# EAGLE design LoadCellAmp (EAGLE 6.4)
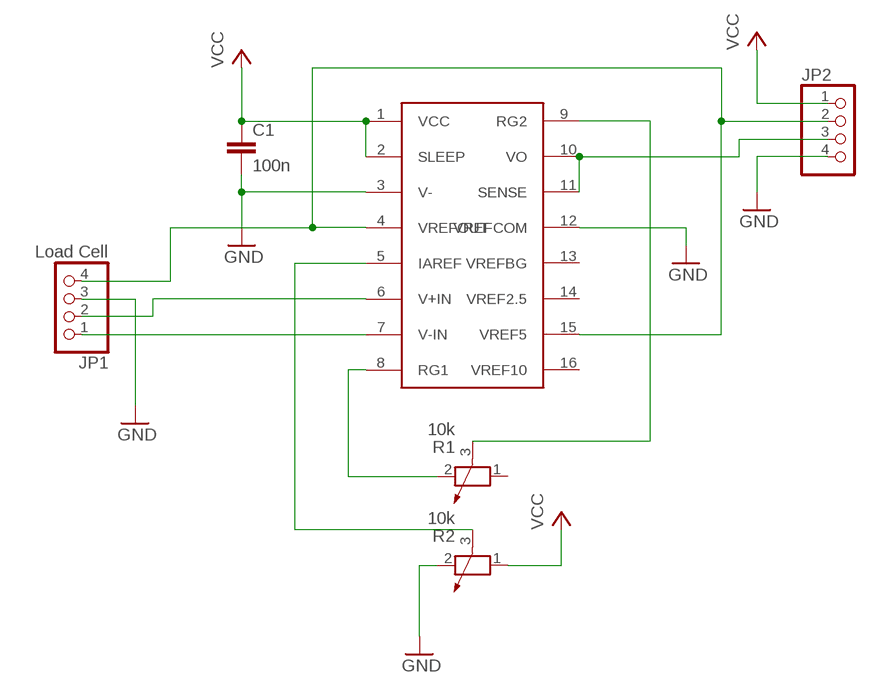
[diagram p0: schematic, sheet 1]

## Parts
C1  100n  C-EUC0603  [C0603]
JP1  Load Cell  PINHD-1X4  [1X04]
JP2  PINHD-1X4  [1X04]
R1  10k  POTENTIOMETER_PT_SPIN  [PT-SPIN]
R2  10k  POTENTIOMETER_PT_SPIN  [PT-SPIN]
U$1  INA125SMD  [SOIC16N]

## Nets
GND: C1.2 JP1.3 JP2.4 R2.2 U$1.3(V-) U$1.12(VREFCOM)
N$1: R1.2 U$1.8(RG1)
N$2: R1.3 U$1.9(RG2)
N$7: JP1.4 JP2.2 U$1.4(VREFOUT) U$1.15(VREF5)
N$8: R2.3 U$1.5(IAREF)
N$10: JP2.3 U$1.10(VO) U$1.11(SENSE)
S+: JP1.2 U$1.6(V+IN)
S-: JP1.1 U$1.7(V-IN)
VCC: C1.1 JP2.1 R2.1 U$1.1(VCC) U$1.2(SLEEP)
Unconnected: R1.1 U$1.13(VREFBG) U$1.14(VREF2.5) U$1.16(VREF10)

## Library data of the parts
C1 = rcl:C-EU: CAPACITOR, European symbol
JP1 JP2 = pinhead:PINHD-1X4: PIN HEADER
R1 R2 = rcl:POTENTIOMETER_: Potentiometer
U$1 = INA125SMD:INA125SMD

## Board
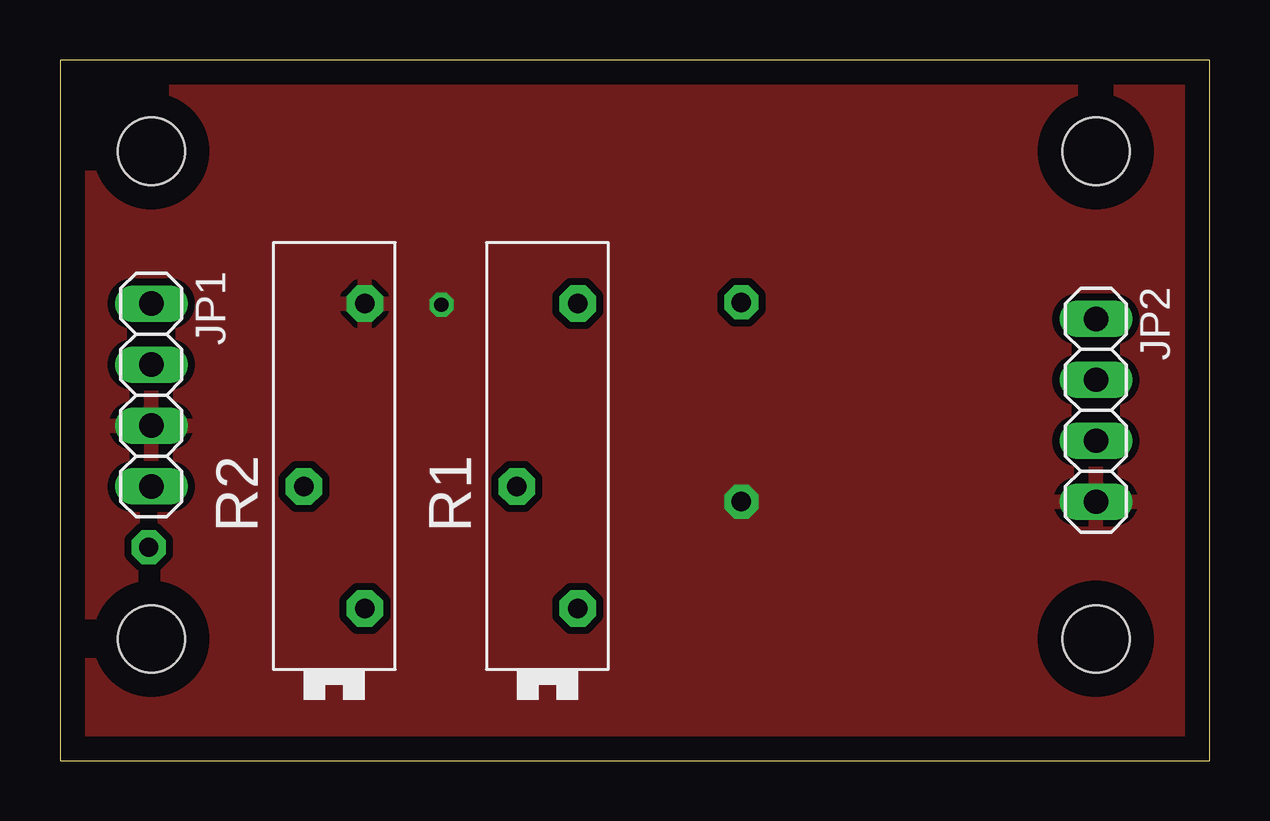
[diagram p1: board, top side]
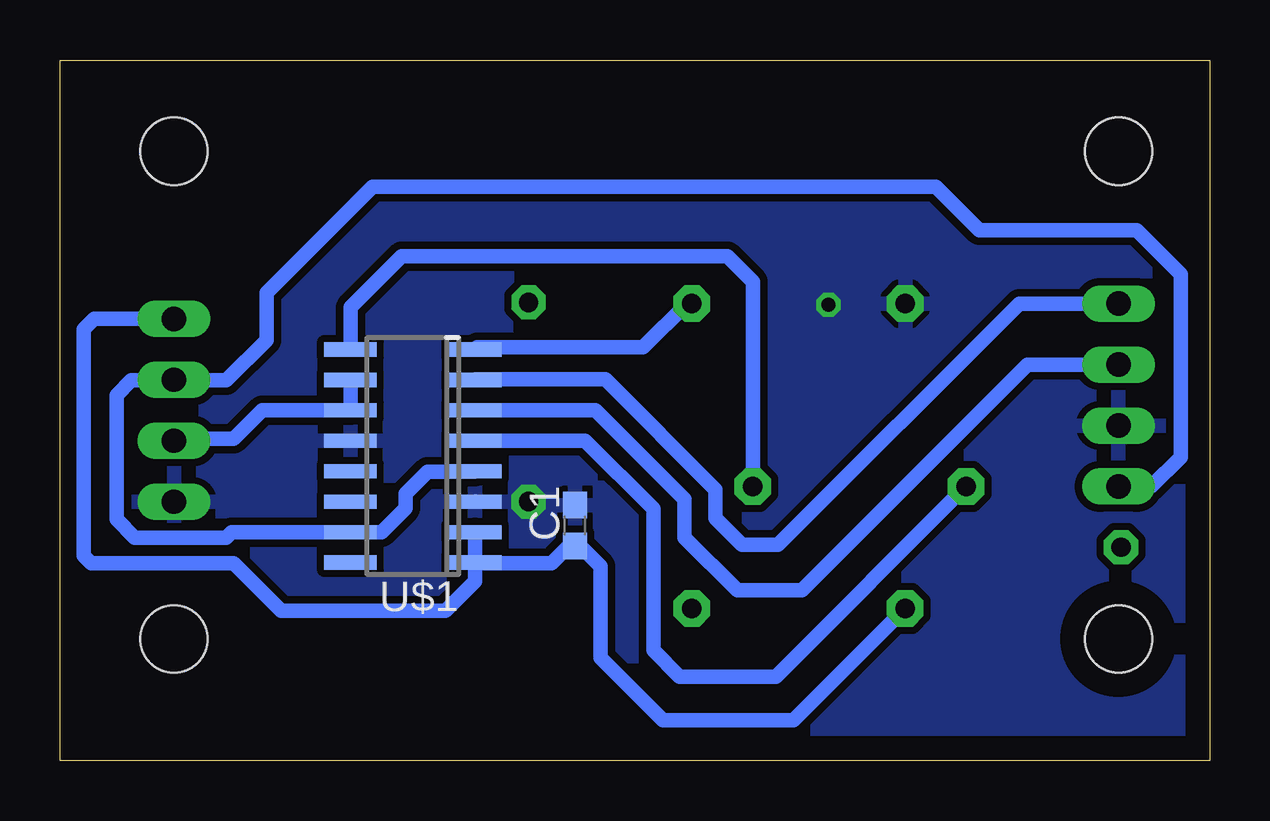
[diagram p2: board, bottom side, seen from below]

Size 47.93 x 29.2 mm. Coordinates in mm from the lower left corner, seen from the top.
Outline: 0,0 47.93,0 47.93,29.2 0,29.2 0,0
Copper layers (1*16): Top 0.035mm / dielectric 1.5mm / Bottom 0.035mm
Design rules "default": minimum track width 10mil, minimum drill 24mil, track to track 8mil, track to pad 8mil, pad to pad 8mil, via to via 8mil, smd to smd 8mil, copper to edge 40mil, drill to drill 8mil, minimum pad ring 10mil, minimum via ring 8mil, stop-mask expansion 4mil, vias tented up to drill 0mil, thermal gap 10mil
Holes 2.8 mm at 3.81,5.08 3.81,25.4 43.18,25.4 43.18,5.08

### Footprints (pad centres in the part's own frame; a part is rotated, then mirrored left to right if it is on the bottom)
C0603 = smd 1.1 x 1: 1 -0.85,0; 2 0.85,0
1X04 = drill 1.016 long: 1 -3.81,0; 2 -1.27,0; 3 1.27,0; 4 3.81,0
PT-SPIN = drill 0.813 pad 1.524 octagon: 1 -6.35,-1.27; 2 6.35,-1.27; 3 -1.27,1.27
SOIC16N = smd 0.6 x 2.2: 1 -4.445,-2.6; 2 -3.175,-2.6; 3 -1.905,-2.6; 4 -0.635,-2.6; 5 0.635,-2.6; 6 1.905,-2.6; 7 3.175,-2.6; 8 4.445,-2.6; 9 4.445,2.6; 10 3.175,2.6; 11 1.905,2.6; 12 0.635,2.6; 13 -0.635,2.6; 14 -1.905,2.6; 15 -3.175,2.6; 16 -4.445,2.6

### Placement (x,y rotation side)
C1  26.47,9.8 90 bottom
JP1  3.81,15.24 270 top
JP2  43.18,14.61 270 top
R1  20.32,12.7 90 top
R2  11.43,12.7 90 top
U$1  33.22,12.7 90 bottom

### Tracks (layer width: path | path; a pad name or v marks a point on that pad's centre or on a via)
GND  (via drill 0.6, 0.8 pad 1.42)
  Bottom 0.61: C1.2 26.5,10.65 26.67,10.82 | 30.6,10.82 U$1.3
  other vias: 28.4,10.8 15.9,19
  pour Bottom (isolate 0.305): 0,0 48.26,0 48.26,30.48 0,30.48
  pour Top (isolate 0.305): 50.8,0 0,0 0,30.48 50.8,30.48
N$1
  Bottom 0.61: R1.2 21.79,19.05 23.62,17.22 30.55,17.22 U$1.8
N$2
  Bottom 0.61: R1.3 19.05,19.96 20.12,21.03 33.68,21.03 35.81,18.9 35.81,17.15 U$1.9
N$3  (via drill 0.8 pad 1.42)
  other vias: 28.4,19.1
N$4  (via drill 0.8 pad 1.42)
  other vias: 3.7,8.9
N$7
  Bottom 0.61: U$1.4 30.65,12.04 32.61,12.04 33.53,11.12 33.53,10.52 34.52,9.53 U$1.15 40.77,9.53 41,9.3 44.81,9.3 45.57,10.06 45.57,15.24 44.96,15.85 43.2,15.85 JP2.2 43.16,15.85 41,15.85 39.32,17.53 39.32,19.51 34.9,23.93 11.43,23.93 9.6,22.1 3.05,22.1 1.22,20.27 1.22,12.65 2.44,11.43 JP1.4
N$8
  Bottom 0.61: U$1.5 26.04,13.34 23.2,10.5 23.2,4.6 22.1,3.5 18.09,3.5 R2.3
N$10
  Bottom 0.61: U$1.10 U$1.11 39.5,14.61 40.69,13.41 43.1,13.41 JP2.3
S+
  Bottom 0.61: U$1.6 25.61,14.61 21.9,10.9 21.9,9.3 19.7,7.1 17,7.1 7.6,16.5 JP1.2
S-
  Bottom 0.61: JP1.1 7.95,19.05 18,9 19.5,9 20.6,10.1 20.6,11.3 25.2,15.9 30.6,15.9 U$1.7
VCC
  Bottom 0.61: JP2.1 46.51,18.41 46.94,17.98 46.94,8.53 46.63,8.23 40.69,8.23 38.71,6.25 31.85,6.25 30.62,7.48 U$1.1 | U$1.1 30.6,8.23 27.43,8.23 26.71,8.95 C1.1 26.25,8.95 25.4,8.1 25.4,4.3 22.8,1.7 17.35,1.7 R2.1 | U$1.2 U$1.1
